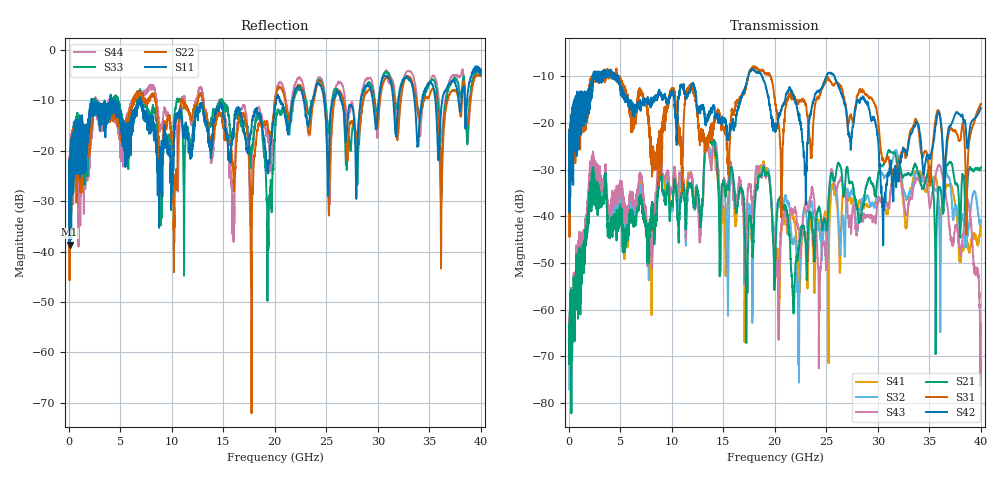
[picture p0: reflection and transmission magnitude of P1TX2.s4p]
!Agilent Technologies,N5245A,MY49151084,A.09.20.08
!Agilent N5245A: A.09.20.08
!Date: Thursday, March 01, 2012 11:50:01
!Correction: S11(Full 4 Port(1,2,3,4))
!S12(Full 4 Port(1,2,3,4))
!S13(Full 4 Port(1,2,3,4))
!S14(Full 4 Port(1,2,3,4))
!S21(Full 4 Port(1,2,3,4))
!S22(Full 4 Port(1,2,3,4))
!S23(Full 4 Port(1,2,3,4))
!S24(Full 4 Port(1,2,3,4))
!S31(Full 4 Port(1,2,3,4))
!S32(Full 4 Port(1,2,3,4))
!S33(Full 4 Port(1,2,3,4))
!S34(Full 4 Port(1,2,3,4))
!S41(Full 4 Port(1,2,3,4))
!S42(Full 4 Port(1,2,3,4))
!S43(Full 4 Port(1,2,3,4))
!S44(Full 4 Port(1,2,3,4))
!S4P File: Measurements: <S11,S12,S13,S14>,
!<S21,S22,S23,S24>,
!<S31,S32,S33,S34>,
!<S41,S42,S43,S44>:
# Hz S  dB  R 50
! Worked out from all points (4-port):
!   3996 points, 50 MHz to 40 GHz, reference 50 ohm
!   strongest paths, dB at 50 MHz, 10.04 GHz, 20.03 GHz, 30.02 GHz, 40 GHz:
!     S42: -27.1, -13.6, -21.8, -23.8, -16.8
!     S31: -25.4, -12.8, -15.4, -19.0, -15.9
!     S21: -65.0, -36.9, -51.3, -31.3, -29.6
!     S43: -61.9, -34.1, -50.3, -36.3, -63.0
!     S32: -77.1, -37.5, -43.4, -31.3, -40.9
!     S41: -63.9, -33.9, -51.5, -36.7, -42.0
!   lowest |S11| = -38.6 dB at 90 MHz (marker M1), VSWR 1.02, Z = 51 + j0.683 ohm
!   |S11| at or under -10 dB: start of sweep to 2.229 GHz; 4.411 GHz to 6.809 GHz (2.398 GHz wide, 42.8 % of centre); 7.003 GHz to 20.14 GHz (13.13 GHz wide, 96.8 % of centre)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
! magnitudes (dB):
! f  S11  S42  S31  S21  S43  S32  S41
! 50 MHz  -24.3  -27.1  -25.4  -65.0  -61.9  -77.1  -63.9
! 90 MHz  -38.6  -39.3  -44.5  -66.0  -66.4  -68.4  -65.5
! 2.25 GHz  -11.6  -13.3  -11.1  -30.7  -27.2  -30.3  -27.9
! 14.17 GHz  -13.1  -17.3  -19.8  -24.6  -24.4  -24.2  -25.8
! 21.79 GHz  -9.9  -14.0  -13.7  -58.0  -39.2  -46.0  -40.5
! 35.98 GHz  -17.6  -18.2  -17.8  -34.0  -29.1  -43.1  -38.8
! 40 GHz  -4.9  -16.8  -15.9  -29.6  -63.0  -40.9  -42.0
